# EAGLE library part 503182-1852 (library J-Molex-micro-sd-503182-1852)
Conn Micro SD Card M 8 POS 1.09mm Solder RA SMD Embossed T/R 0.5A/Contact
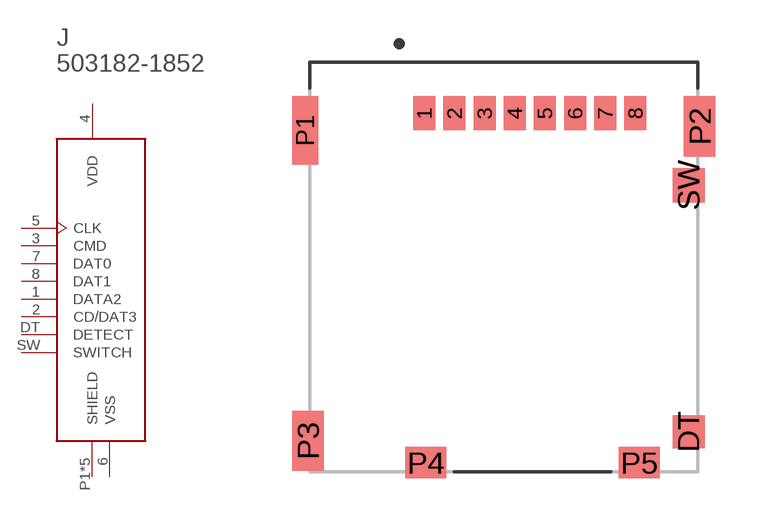
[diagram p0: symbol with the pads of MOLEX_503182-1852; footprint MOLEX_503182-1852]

Designator prefix J

## 503182-1852 (DESCRIPTION: MICRO SD NORMAL ULTRALOWPRO8CKTE; DIGI-KEY_PART_NUMBER: WM12834CT-ND; DIGI-KEY_PURCHASE_URL: https://www.digikey.com/product-detail/en/molex/5031821852/WM12834CT-ND/5823232?utm_source=snapeda&utm_medium=aggregator&utm_campaign=symbol; MF: Molex; MP: 5031821852; PACKAGE: None)  [MOLEX_503182-1852]
1  DATA2
2  CD/DAT3
3  CMD
4  VDD  pwr
5  CLK
6  VSS  pwr
7  DAT0
8  DAT1
DT  DETECT
P1  SHIELD  pas
P2  SHIELD  pas
P3  SHIELD  pas
P4  SHIELD  pas
P5  SHIELD  pas
SW  SWITCH

## Footprint MOLEX_503182-1852 (pad centres in mm)
smd 0.8 x 1.24: 1 -2.9,6.355; 2 -1.8,6.355; 3 -0.7,6.355; 4 0.4,6.355; 5 1.5,6.355; 6 2.6,6.355; 7 3.7,6.355; 8 4.8,6.355
smd 1.16 x 1.2: DT 6.74,-5.275
smd 0.95 x 2.5: P1 -7.245,5.725
smd 1.15 x 2.2: P2 7.145,5.875; P3 -7.145,-5.605
smd 1.5 x 1.15: P4 -2.84,-6.4; P5 4.94,-6.4
smd 1.16 x 1.25: SW 6.74,3.725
